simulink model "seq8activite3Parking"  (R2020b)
settings: Solver=VariableStepAuto  StartTime=0.0  StopTime=inf  RelTol=1e-3  EnableMultiTasking=on
libraries: sldrtlib x1

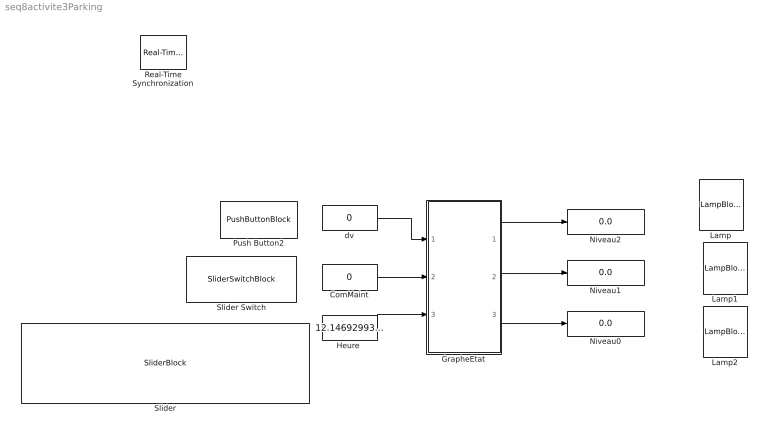
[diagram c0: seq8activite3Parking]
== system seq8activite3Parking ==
  ComMaint : Constant  Value=0
  GrapheEtat : Stateflow chart  TreatAsAtomicUnit=on
  "Heure " : Constant  Value=12.14692993164062
  Lamp : LampBlock
  Lamp1 : LampBlock
  Lamp2 : LampBlock
  Niveau0 : Display
  Niveau1 : Display
  Niveau2 : Display
  Push Button2 : PushButtonBlock  LabelPosition=Top
  Real-Time Synchronization : sldrtlib/Real-Time Synchronization  SampleTime=0.1  MaxMissedTicks=10  ShowMissedTicks=off  YieldWhenWaiting=off
  Slider : SliderBlock  ScaleMax=23.9
  Slider Switch : SliderSwitchBlock
  dv : Constant  Value=0
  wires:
  GrapheEtat/3(LED0) -> Niveau0/1
  dv/1 -> GrapheEtat/1(DV)
  ComMaint/1 -> GrapheEtat/2(ComMaint)
  "Heure "/1 -> GrapheEtat/3(Heure)
  GrapheEtat/2(LED1) -> Niveau1/1
  GrapheEtat/1(LED2) -> Niveau2/1

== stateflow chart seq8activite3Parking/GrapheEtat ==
  state nuit
  state Maintenance
  state jour
    state pasVoiture
    state voitureN1
    (default) -> pasVoiture
    pasVoiture -> voitureN1
    voitureN1 -> pasVoiture
  nuit -> Maintenance
  (default) -> nuit
  Maintenance -> nuit
  jour -> nuit
  nuit -> jour
  jour -> Maintenance
  Maintenance -> jour
  data: LED2 output; LED1 output; LED0 output; DV input; ComMaint input; Heure input
